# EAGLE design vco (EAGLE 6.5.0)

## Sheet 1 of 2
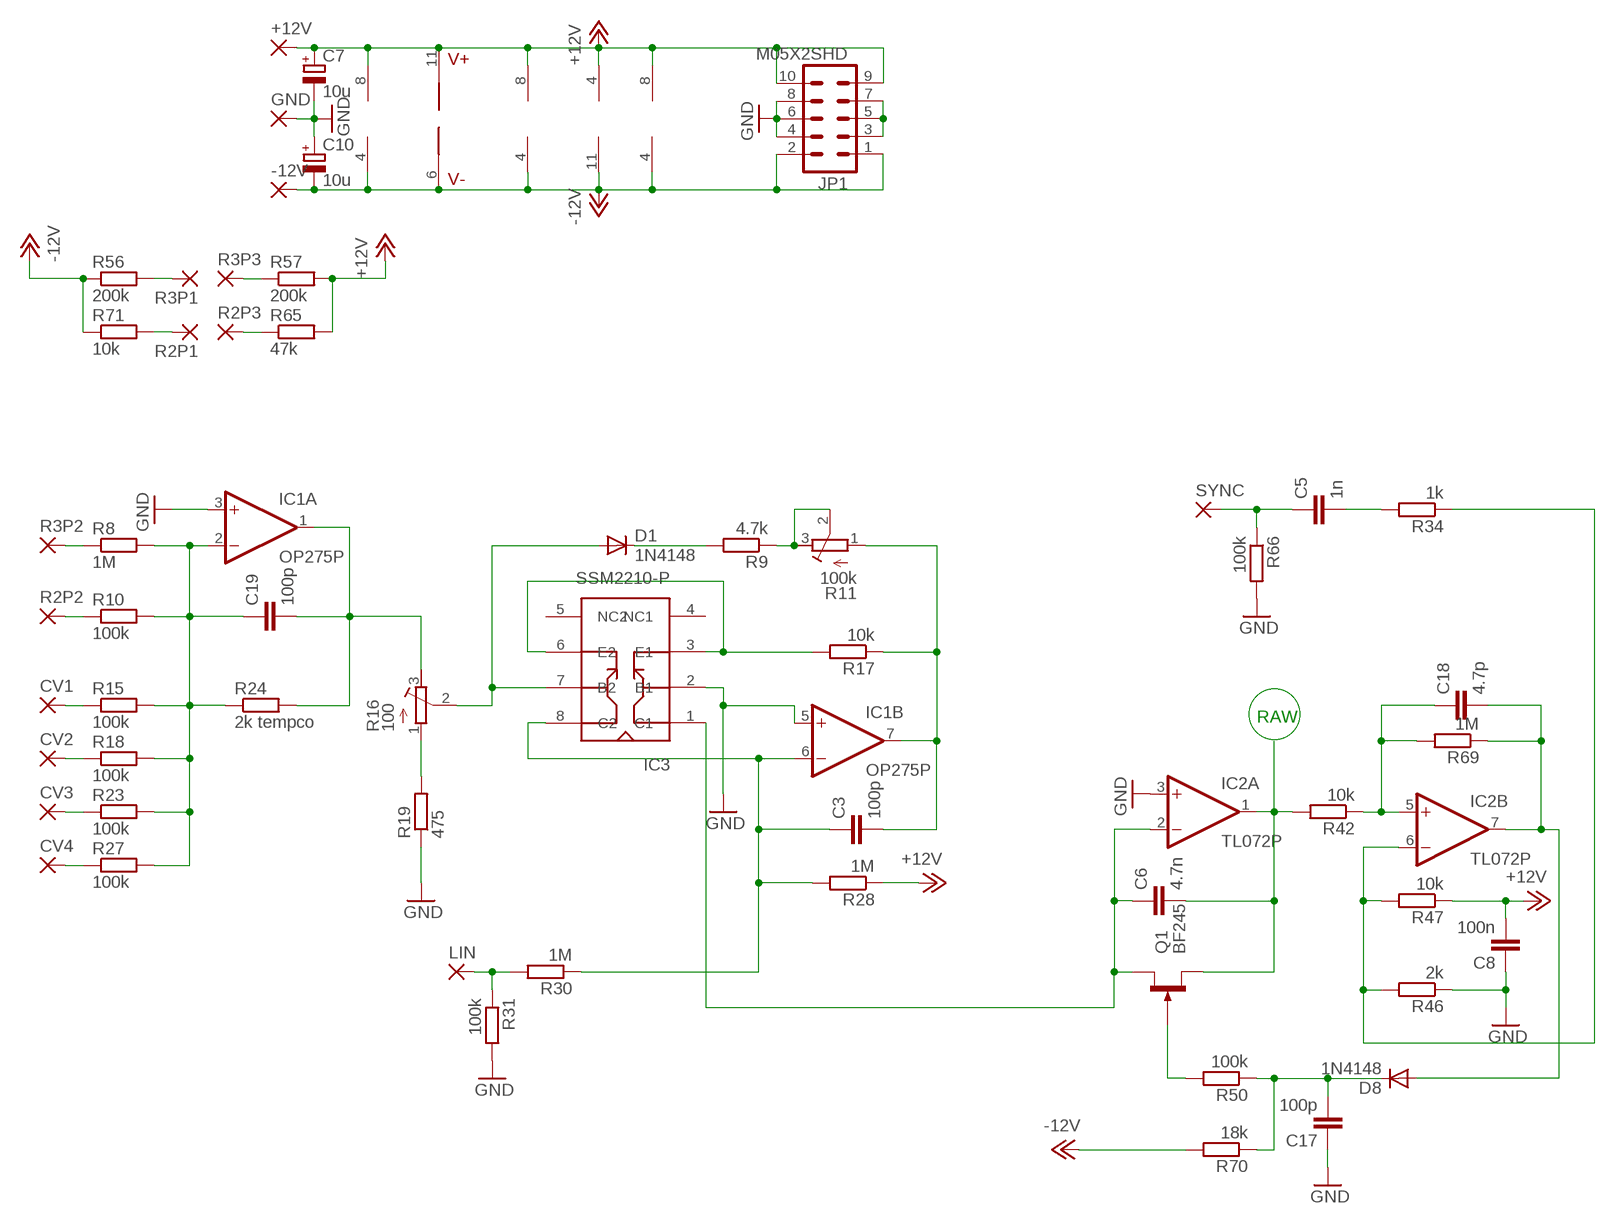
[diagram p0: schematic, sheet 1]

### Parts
+12V  2,54/1,0  [2,54/1,0]
-12V  2,54/1,0  [2,54/1,0]
C3  100p  C-EU102-043X133  [C102-043X133]
C5  1n  C-EU102-043X133  [C102-043X133]
C6  4.7n  C-EU102-043X133  [C102-043X133]
C7  10u  CPOL-EUE2.5-7  [E2,5-7]
C8  100n  C-EU102-043X133  [C102-043X133]
C10  10u  CPOL-EUE2.5-7  [E2,5-7]
C17  100p  C-EU102-043X133  [C102-043X133]
C18  4.7p  C-EU102-043X133  [C102-043X133]
C19  100p  C-EU102-043X133  [C102-043X133]
CV1  2,54/1,0  [2,54/1,0]
CV2  2,54/1,0  [2,54/1,0]
CV3  2,54/1,0  [2,54/1,0]
CV4  2,54/1,0  [2,54/1,0]
D1  1N4148  1N4148DO35-7  [DO35-7]
D8  1N4148  1N4148DO35-7  [DO35-7]
GND  2,54/1,0  [2,54/1,0]
IC1  OP275P  [DIL08]
IC2  TL072P  [DIL08]
IC3  SSM2210-P  [DIL08]
IC4  TL074P  [DIL14]
IC5  LM13700N  [DIL16]
IC6  TL072P  [DIL08]
JP1  M05X2SHD  [2X5-SHROUDED]
LIN  2,54/1,0  [2,54/1,0]
Q1  BF245  [SOT54C]
R2P1  2,54/1,0  [2,54/1,0]
R2P2  2,54/1,0  [2,54/1,0]
R2P3  2,54/1,0  [2,54/1,0]
R3P1  2,54/1,0  [2,54/1,0]
R3P2  2,54/1,0  [2,54/1,0]
R3P3  2,54/1,0  [2,54/1,0]
R8  1M  R-EU_0309/10  [0309/10]
R9  4.7k  R-EU_0309/10  [0309/10]
R10  100k  R-EU_0309/10  [0309/10]
R11  100k  R-TRIMM64W  [RTRIM64W]
R15  100k  R-EU_0309/10  [0309/10]
R16  100  R-TRIMM64W  [RTRIM64W]
R17  10k  R-EU_0309/10  [0309/10]
R18  100k  R-EU_0309/10  [0309/10]
R19  475  R-EU_0309/10  [0309/10]
R23  100k  R-EU_0309/10  [0309/10]
R24  2k tempco  R-EU_0309/12  [0309/12]
R27  100k  R-EU_0309/10  [0309/10]
R28  1M  R-EU_0309/10  [0309/10]
R30  1M  R-EU_0309/10  [0309/10]
R31  100k  R-EU_0309/10  [0309/10]
R34  1k  R-EU_0309/10  [0309/10]
R42  10k  R-EU_0309/10  [0309/10]
R46  2k  R-EU_0309/10  [0309/10]
R47  10k  R-EU_0309/10  [0309/10]
R50  100k  R-EU_0309/10  [0309/10]
R56  200k  R-EU_0309/10  [0309/10]
R57  200k  R-EU_0309/10  [0309/10]
R65  47k  R-EU_0309/10  [0309/10]
R66  100k  R-EU_0309/10  [0309/10]
R69  1M  R-EU_0309/10  [0309/10]
R70  18k  R-EU_0309/10  [0309/10]
R71  10k  R-EU_0309/10  [0309/10]
SYNC  2,54/1,0  [2,54/1,0]

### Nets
+12V: +12V.1(P) C7.+ C8.2 IC1.8(P:V+) IC2.8(P:V+) IC4.4(P:V+) IC5.11(V+) IC6.8(P:V+) JP1.9 JP1.10 R28.1 R47.1 R57.2 R65.2 ; also sheet 2
-12V: -12V.1(P) C10.- IC1.4(P:V-) IC2.4(P:V-) IC4.11(P:V-) IC5.6(V-) IC6.4(P:V-) JP1.1 JP1.2 R56.1 R70.2 R71.1 ; also sheet 2
GND: C7.- C8.1 C10.+ C17.1 GND.1(P) IC1.3(A:+IN) IC1.5(B:+IN) IC2.3(A:+IN) IC3.2(B1) JP1.4 JP1.6 JP1.8 R19.1 R31.2 R46.1 R66.2 ; also sheet 2
N$1: R3P1.1(P) R56.2
N$2: R2P1.1(P) R71.2
N$3: R2P3.1(P) R65.1
N$4: R3P3.1(P) R57.1
N$5: R3P2.1(P) R8.1
N$6: R2P2.1(P) R10.1
N$7: CV1.1(P) R15.1
N$8: CV2.1(P) R18.1
N$9: CV3.1(P) R23.1
N$10: CV4.1(P) R27.1
N$11: C19.1 IC1.2(A:-IN) R8.2 R10.2 R15.2 R18.2 R23.2 R24.1 R27.2
N$12: C19.2 IC1.1(A:OUT) R16.3(E) R24.2
N$13: Q1.G R50.2
N$14: R16.1(A) R19.2
N$15: LIN.1(P) R30.2 R31.1
N$16: C3.1 IC1.6(B:-IN) IC3.8(C2) R28.2 R30.1
N$17: C3.2 IC1.7(B:OUT) R11.1(A) R17.1
N$18: IC3.3(E1) IC3.6(E2) R17.2
N$19: C17.2 D8.C R50.1 R70.1
N$20: C6.1 IC2.2(A:-IN) IC3.1(C1) Q1.D
N$22: D1.A IC3.7(B2) R16.2(S)
N$23: D1.C R9.2
N$24: R9.1 R11.2(S) R11.3(E)
N$25: C18.1 IC2.5(B:+IN) R42.1 R69.2
N$26: C18.2 D8.A IC2.7(B:OUT) R69.1
N$27: IC2.6(B:-IN) R34.1 R46.2 R47.2
N$28: C5.2 R34.2
N$29: C5.1 R66.1 SYNC.1(P)
N$64: JP1.3 JP1.5 JP1.7
RAW: C6.2 IC2.1(A:OUT) Q1.S R42.2 ; also sheet 2
Unconnected: IC3.4(NC1) IC3.5(NC2)

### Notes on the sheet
- RAW

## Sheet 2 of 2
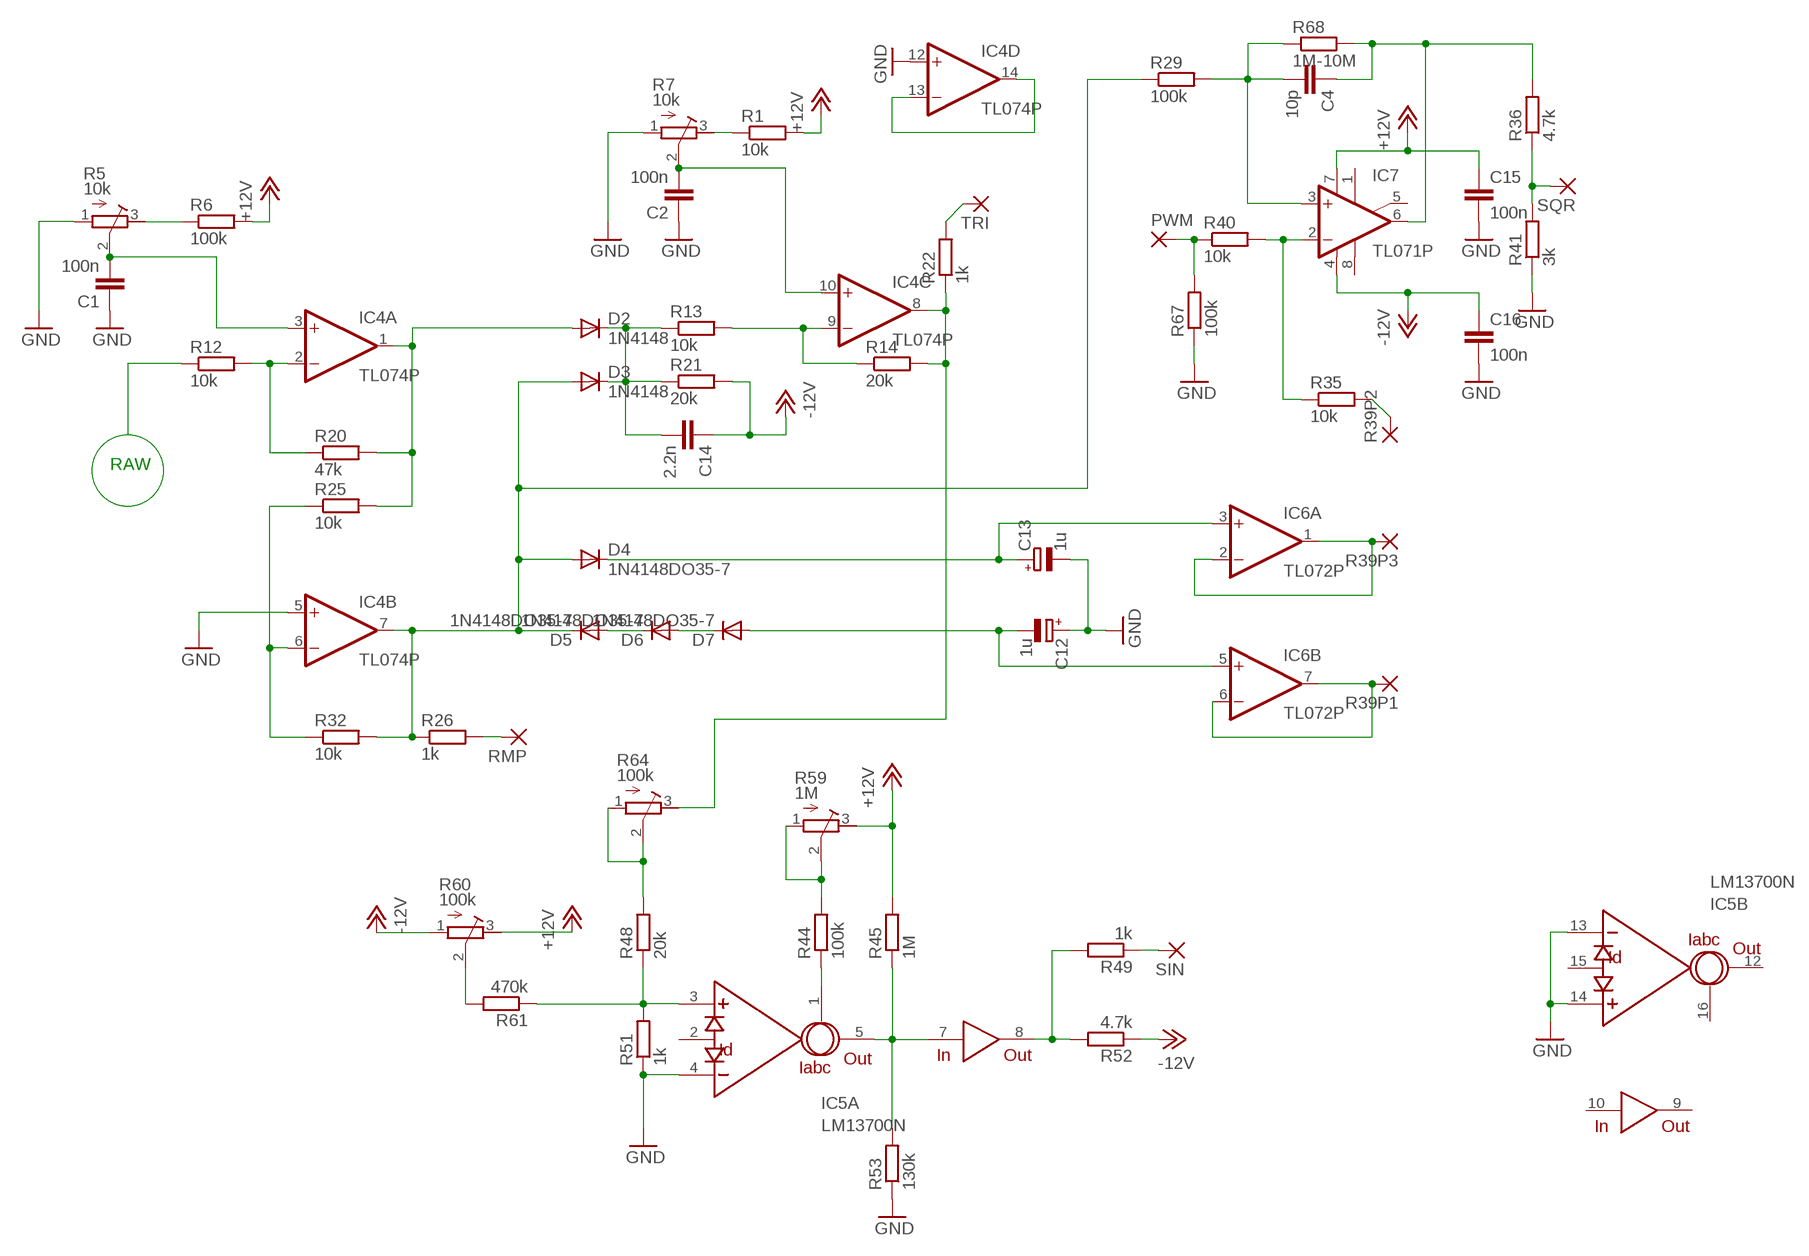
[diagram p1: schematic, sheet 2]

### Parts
C1  100n  C-EU102-043X133  [C102-043X133]
C2  100n  C-EU102-043X133  [C102-043X133]
C4  10p  C-EU102-043X133  [C102-043X133]
C12  1u  CPOL-EUE2.5-7  [E2,5-7]
C13  1u  CPOL-EUE2.5-7  [E2,5-7]
C14  2.2n  C-EU102-043X133  [C102-043X133]
C15  100n  C-EU050-035X075  [C050-035X075]
C16  100n  C-EU050-035X075  [C050-035X075]
D2  1N4148  1N4148DO35-7  [DO35-7]
D3  1N4148  1N4148DO35-7  [DO35-7]
D4  1N4148DO35-7  [DO35-7]
D5  1N4148DO35-7  [DO35-7]
D6  1N4148DO35-7  [DO35-7]
D7  1N4148DO35-7  [DO35-7]
IC7  TL071P  [DIL08]
PWM  2,54/1,0  [2,54/1,0]
R1  10k  R-EU_0309/10  [0309/10]
R5  10k  R-TRIMM64W  [RTRIM64W]
R6  100k  R-EU_0309/10  [0309/10]
R7  10k  R-TRIMM64W  [RTRIM64W]
R12  10k  R-EU_0309/10  [0309/10]
R13  10k  R-EU_0309/10  [0309/10]
R14  20k  R-EU_0309/10  [0309/10]
R20  47k  R-EU_0309/10  [0309/10]
R21  20k  R-EU_0309/10  [0309/10]
R22  1k  R-EU_0309/10  [0309/10]
R25  10k  R-EU_0309/10  [0309/10]
R26  1k  R-EU_0309/10  [0309/10]
R29  100k  R-EU_0309/10  [0309/10]
R32  10k  R-EU_0309/10  [0309/10]
R35  10k  R-EU_0309/10  [0309/10]
R36  4.7k  R-EU_0309/10  [0309/10]
R39P1  2,54/1,0  [2,54/1,0]
R39P2  2,54/1,0  [2,54/1,0]
R39P3  2,54/1,0  [2,54/1,0]
R40  10k  R-EU_0309/10  [0309/10]
R41  3k  R-EU_0309/10  [0309/10]
R44  100k  R-EU_0309/10  [0309/10]
R45  1M  R-EU_0309/10  [0309/10]
R48  20k  R-EU_0309/10  [0309/10]
R49  1k  R-EU_0309/10  [0309/10]
R51  1k  R-EU_0309/10  [0309/10]
R52  4.7k  R-EU_0309/10  [0309/10]
R53  130k  R-EU_0309/10  [0309/10]
R59  1M  R-TRIMM64W  [RTRIM64W]
R60  100k  R-TRIMM64W  [RTRIM64W]
R61  470k  R-EU_0309/10  [0309/10]
R64  100k  R-TRIMM64W  [RTRIM64W]
R67  100k  R-EU_0309/10  [0309/10]
R68  1M-10M  R-EU_0309/10  [0309/10]
RMP  2,54/1,0  [2,54/1,0]
SIN  2,54/1,0  [2,54/1,0]
SQR  2,54/1,0  [2,54/1,0]
TRI  2,54/1,0  [2,54/1,0]

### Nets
+12V: C15.1 IC7.7(V+) R1.2 R6.2 R45.2 R59.3(E) R60.3(E) ; also sheet 1
-12V: C14.1 C16.1 IC7.4(V-) R21.2 R52.1 R60.1(A) ; also sheet 1
GND: C1.1 C2.1 C12.+ C13.- C15.2 C16.2 IC4.5(B:+IN) IC4.12(D:+IN) IC5.4(A:-IN) IC5.13(B:-IN) IC5.14(B:+IN) R5.1(A) R7.1(A) R41.1 R51.1 R53.1 R67.1 ; also sheet 1
N$21: C2.2 IC4.10(C:+IN) R7.2(S)
N$30: R1.1 R7.3(E)
N$31: R26.2 RMP.1(P)
N$32: R5.3(E) R6.1
N$33: C1.2 IC4.3(A:+IN) R5.2(S)
N$34: IC4.2(A:-IN) R12.2 R20.1
N$35: D2.A IC4.1(A:OUT) R20.2 R25.2
N$36: IC4.6(B:-IN) R25.1 R32.1
N$37: IC4.13(D:-IN) IC4.14(D:OUT)
N$38: D5.A D6.C
N$39: C14.2 D2.C D3.C R13.1 R21.1
N$40: D3.A D4.A D5.C IC4.7(B:OUT) R26.1 R29.1 R32.2
N$41: IC4.9(C:-IN) R13.2 R14.1
N$42: IC4.8(C:OUT) R14.2 R22.1 R64.3(E)
N$43: R22.2 TRI.1(P)
N$44: D6.A D7.C
N$45: C13.+ D4.C IC6.3(A:+IN)
N$46: C12.- D7.A IC6.5(B:+IN)
N$47: R60.2(S) R61.2
N$48: R35.2 R39P2.1(P)
N$49: R36.1 R41.2 SQR.1(P)
N$50: IC7.2(-IN) R35.1 R40.2
N$51: PWM.1(P) R40.1 R67.2
N$52: C4.2 IC7.3(+IN) R29.2 R68.1
N$53: C4.1 IC7.6(OUT) R36.2 R68.2
N$54: IC5.3(A:+IN) R48.1 R51.2 R61.1
N$56: R48.2 R64.1(A) R64.2(S)
N$57: IC6.1(A:OUT) IC6.2(A:-IN) R39P3.1(P)
N$58: IC6.6(B:-IN) IC6.7(B:OUT) R39P1.1(P)
N$59: IC5.5(A:OUT) IC5.7(IN) R45.1 R53.2
N$60: IC5.1(A:IABC) R44.1
N$61: IC5.8(OUT) R49.2 R52.2
N$62: R44.2 R59.1(A) R59.2(S)
N$63: R49.1 SIN.1(P)
RAW: R12.1 ; also sheet 1
Unconnected: IC5.2(A:ID) IC5.9(OUT) IC5.10(IN) IC5.12(B:OUT) IC5.15(B:ID) IC5.16(B:IABC) IC7.1(ON1) IC7.5(ON2) IC7.8(OPT)

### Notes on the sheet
- RAW

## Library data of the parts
+12V -12V CV1-CV4 GND LIN PWM R2P1-R2P3 R3P1-R3P3 R39P1-R39P3 RMP SIN SQR SYNC TRI = wirepad:2,54/1,0: THROUGH-HOLE PAD
C1-C6 C8 C14-C19 = rcl:C-EU: CAPACITOR, European symbol
C7 C10 C12 C13 = rcl:CPOL-EU: POLARIZED CAPACITOR, European symbol
D1-D8 = diode:1N4148: DIODE
IC1 = linear:OP275: Dual Very Low Noise Precision Operational Amplifier Source: http://www.analog.com/static/imported-files/data_sheets/OP270.pdf
IC2 IC6 = linear:TL072: OP AMP
IC3 = cavalier:SSM2210
IC4 = linear:TL074: OP AMP
IC5 = synthdiy:LM13700: National Dual OTA with buffers.
IC7 = linear:TL071: OP AMP
JP1 = SparkFun:M05X2: Header 5x2 Standard 10-pin dual row 0.1" header. Commonly used with AVR-ISP. Use with Spark Fun Electronics SKU: PRT-00778
Q1 = transistor-small-signal:BF245: N-CHANNEL FET http://www.onsemi.com/pub/Collateral/BF245A-D.PDF
R1 R6 R8-R10 R12-R15 R17-R32 R34-R36 R40-R42 R44-R53 R56 R57 R61 R65-R71 = rcl:R-EU_: RESISTOR, European symbol
R5 R7 R11 R16 R59 R60 R64 = rcl:R-TRIMM: Trimm resistor

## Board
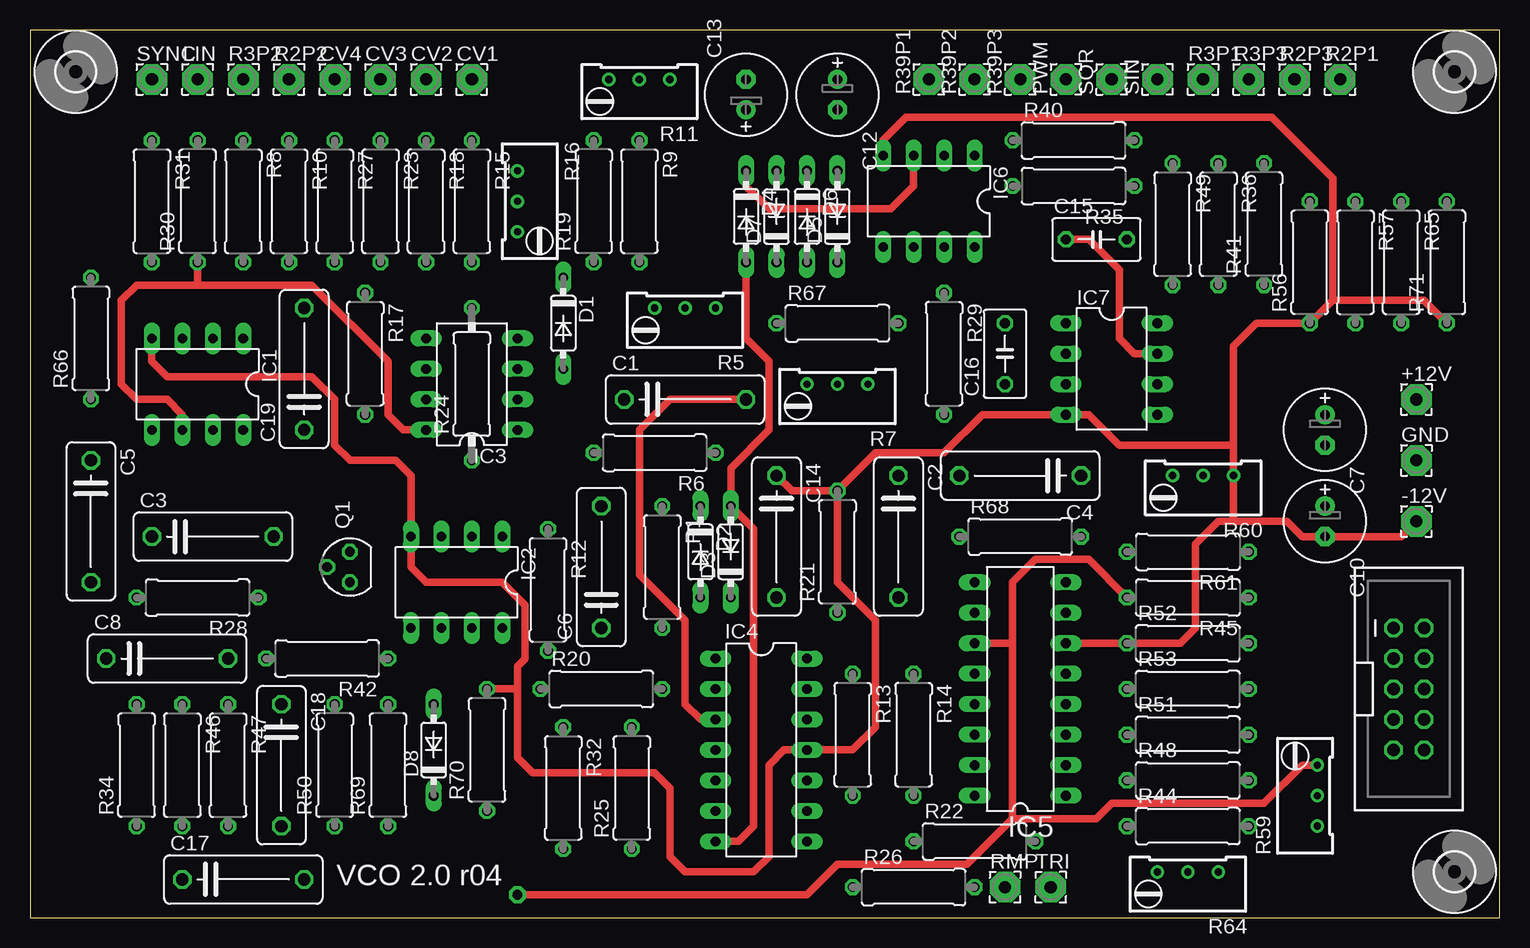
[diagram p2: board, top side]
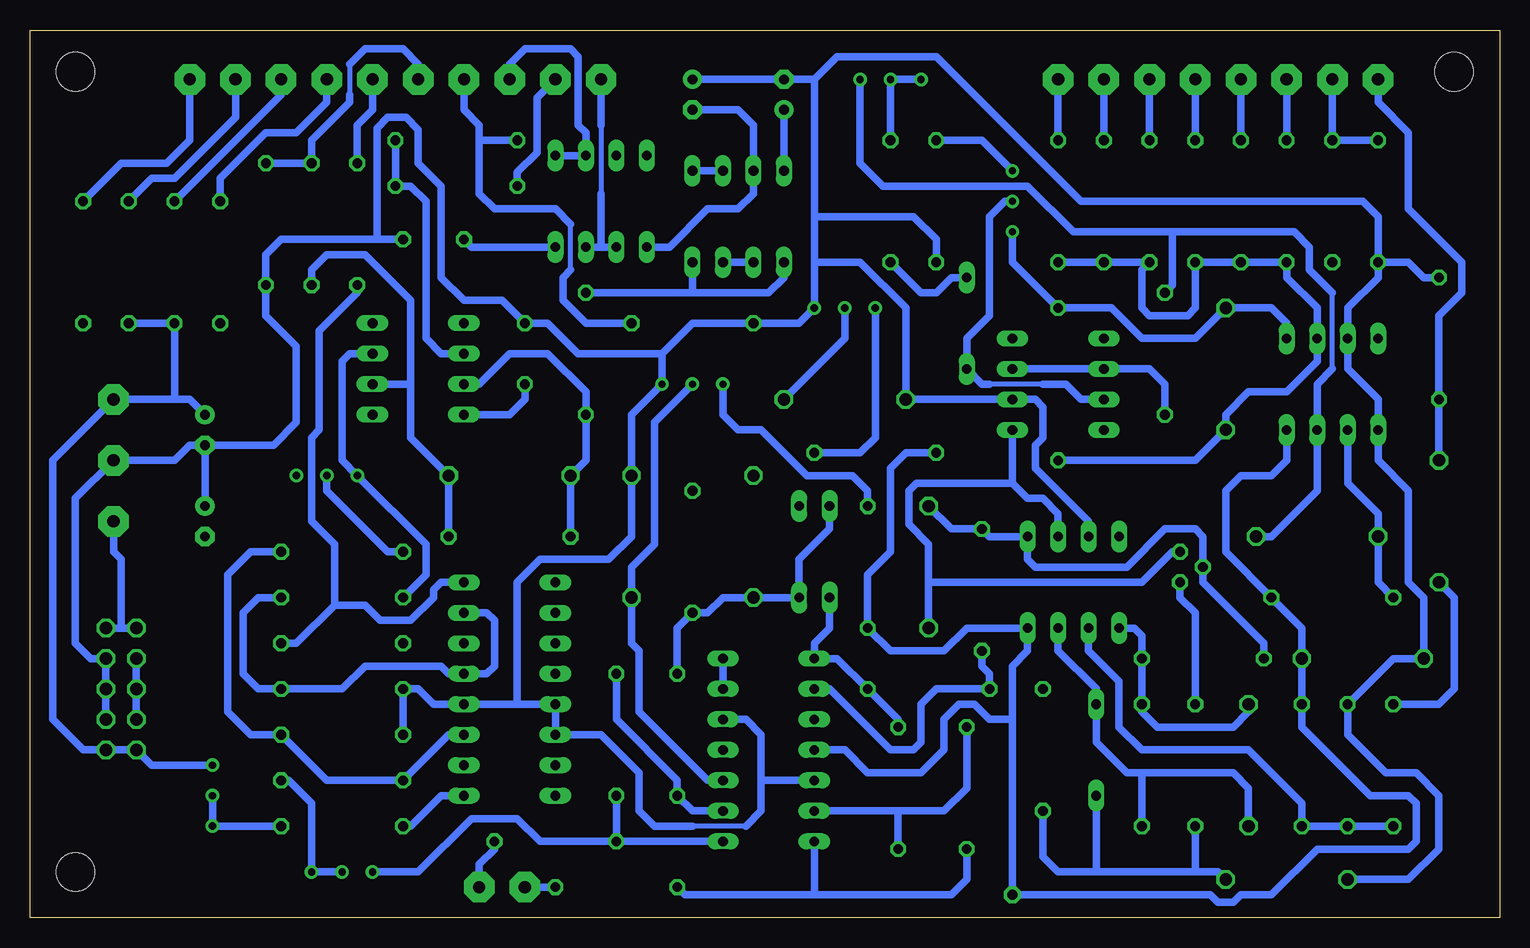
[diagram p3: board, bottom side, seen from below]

Size 122.53 x 73.97 mm. Coordinates in mm from the lower left corner, seen from the top.
Outline: 0,0 122.53,0 122.53,73.97 0,73.97 0,0
Copper layers (1*16): Top 0.035mm / dielectric 1.5mm / Bottom 0.035mm
Design rules "default": minimum track width 10mil, minimum drill 24mil, track to track 8mil, track to pad 8mil, pad to pad 8mil, via to via 8mil, smd to smd 8mil, copper to edge 40mil, drill to drill 8mil, minimum pad ring 10mil, minimum via ring 8mil, stop-mask expansion 4mil, vias tented up to drill 0mil, thermal gap 10mil

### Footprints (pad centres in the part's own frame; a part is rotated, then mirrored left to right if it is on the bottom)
2,54/1,0 = drill 1.016 pad 2.54 octagon: 1 0,0
C102-043X133 = drill 1.016 octagon: 1 -5.08,0; 2 5.08,0
E2,5-7 = drill 0.813 pad 1.6: + -1.27,0 | drill 0.813 pad 1.6 octagon: - 1.27,0
C050-035X075 = drill 0.813 octagon: 1 -2.54,0; 2 2.54,0
DO35-7 = drill 0.813 long: A 3.81,0; C -3.81,0
DIL08 = drill 0.813 pad 1.27 long: 1 -3.81,-3.81; 2 -1.27,-3.81; 3 1.27,-3.81; 4 3.81,-3.81; 5 3.81,3.81; 6 1.27,3.81; 7 -1.27,3.81; 8 -3.81,3.81
DIL14 = drill 0.813 long: 1 -7.62,-3.81; 2 -5.08,-3.81; 3 -2.54,-3.81; 4 0,-3.81; 5 2.54,-3.81; 6 5.08,-3.81; 7 7.62,-3.81; 8 7.62,3.81; 9 5.08,3.81; 10 2.54,3.81; 11 0,3.81; 12 -2.54,3.81; 13 -5.08,3.81; 14 -7.62,3.81
DIL16 = drill 0.813 long: 1 -8.89,-3.81; 2 -6.35,-3.81; 3 -3.81,-3.81; 4 -1.27,-3.81; 5 1.27,-3.81; 6 3.81,-3.81; 7 6.35,-3.81; 8 8.89,-3.81; 9 8.89,3.81; 10 6.35,3.81; 11 3.81,3.81; 12 1.27,3.81; 13 -1.27,3.81; 14 -3.81,3.81; 15 -6.35,3.81; 16 -8.89,3.81
2X5-SHROUDED = drill 1.016 octagon: 1 -1.27,5.08; 2 1.27,5.08; 3 -1.27,2.54; 4 1.27,2.54; 5 -1.27,0; 6 1.27,0; 7 -1.27,-2.54; 8 1.27,-2.54; 9 -1.27,-5.08; 10 1.27,-5.08
SOT54C = drill 0.813 octagon: D 1.27,0; G -1.27,0; S 0,1.905
0309/10 = drill 0.813 octagon: 1 -5.08,0; 2 5.08,0
RTRIM64W = drill 0.61: 1 1.27,-2.54; 2 1.27,0; 3 1.27,2.54
0309/12 = drill 0.813 octagon: 1 -6.35,0; 2 6.35,0
3,2 = hole 3.2: 0,0

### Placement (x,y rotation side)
+12V  115.57,43.18 0 top
-12V  115.57,33.02 0 top
C1  54.61,43.18 0 top
C2  72.39,31.75 270 top
C3  15.24,31.75 0 top
C4  82.55,36.83 180 top
C5  5.08,33.02 270 top
C6  47.62,29.21 90 top
C7  107.95,40.64 270 top
C8  11.43,21.59 0 top
C10  107.95,33.02 270 top
C12  67.31,68.58 270 top
C13  59.69,68.58 90 top
C14  62.23,31.75 270 top
C15  88.9,56.52 0 top
C16  81.28,46.99 90 top
C17  17.78,3.17 0 top
C18  20.95,12.7 270 top
C19  22.86,45.72 90 top
CV1  36.83,69.85 0 top
CV2  33.02,69.85 0 top
CV3  29.21,69.85 0 top
CV4  25.4,69.85 0 top
D1  44.45,49.53 270 top
D2  55.88,30.48 270 top
D3  58.42,30.48 90 top
D4  59.69,58.42 270 top
D5  67.31,58.42 90 top
D6  64.77,58.42 270 top
D7  62.23,58.42 90 top
D8  33.66,13.97 90 top
GND  115.57,38.1 0 top
IC1  13.97,44.45 180 top
IC2  35.56,27.94 180 top
IC3  36.83,44.45 90 top
IC4  60.96,13.97 270 top
IC5  82.55,19.05 90 top
IC6  74.93,59.69 180 top
IC7  90.17,45.72 270 top
JP1  114.94,19.05 0 top
LIN  13.97,69.85 0 top
PWM  86.36,69.85 90 top
Q1  26.67,29.21 90 top
R1  52.7,29.21 270 top
R2P1  109.22,69.85 0 top
R2P2  21.59,69.85 0 top
R2P3  105.41,69.85 0 top
R3P1  97.79,69.85 0 top
R3P2  17.78,69.85 0 top
R3P3  101.6,69.85 0 top
R5  54.61,49.53 90 top
R6  52.07,38.73 180 top
R7  67.31,43.18 90 top
R8  17.78,59.69 270 top
R9  50.8,59.69 270 top
R10  21.59,59.69 270 top
R11  50.8,68.58 90 top
R12  43.18,27.3 270 top
R13  68.58,15.24 270 top
R14  73.66,15.24 270 top
R15  36.83,59.69 270 top
R16  41.91,59.69 180 top
R17  27.94,46.99 270 top
R18  33.02,59.69 270 top
R19  46.99,59.69 90 top
R20  47.62,19.05 0 top
R21  67.31,30.48 90 top
R22  78.74,6.35 0 top
R23  29.21,59.69 270 top
R24  36.83,44.45 90 top
R25  50.16,10.79 90 top
R26  73.66,2.54 0 top
R27  25.4,59.69 270 top
R28  13.97,26.67 180 top
R29  76.2,46.99 270 top
R30  13.97,59.69 90 top
R31  10.16,59.69 270 top
R32  44.45,10.79 270 top
R34  8.89,12.7 90 top
R35  87,60.96 180 top
R36  99.06,57.78 270 top
R39P1  74.93,69.85 90 top
R39P2  78.74,69.85 90 top
R39P3  82.55,69.85 90 top
R40  87,64.77 0 top
R41  102.87,57.78 90 top
R42  24.77,21.59 180 top
R44  96.52,7.62 0 top
R45  96.52,26.67 180 top
R46  12.7,12.7 270 top
R47  16.51,12.7 270 top
R48  96.52,11.43 0 top
R49  95.25,57.78 270 top
R50  25.4,12.7 90 top
R51  96.52,15.24 0 top
R52  96.52,22.86 0 top
R53  96.52,19.05 0 top
R56  106.68,54.61 90 top
R57  110.49,54.61 270 top
R59  106.05,10.16 0 top
R60  97.79,35.56 90 top
R61  96.52,30.48 180 top
R64  96.52,2.54 90 top
R65  114.3,54.61 270 top
R66  5.08,48.26 90 top
R67  67.31,49.53 0 top
R68  82.55,31.75 0 top
R69  29.84,12.7 90 top
R70  38.1,13.97 90 top
R71  118.11,54.61 90 top
RMP  81.28,2.54 0 top
SIN  93.98,69.85 90 top
SQR  90.17,69.85 90 top
SYNC  10.16,69.85 0 top
TRI  85.09,2.54 0 top
U$1  [3,2]  3.81,70.48 0 top
U$2  [3,2]  118.75,70.48 0 top
U$3  [3,2]  118.75,3.81 0 top

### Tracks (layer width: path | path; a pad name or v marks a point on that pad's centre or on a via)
+12V  (via drill 0.8 pad 1.42)
  Top 0.61: 81.92,8.26 78.11,4.45 67.31,4.45 64.77,1.91 v40.64,1.91 | 81.92,22.86 81.92,8.26 | 81.92,8.26 88.9,8.26 90.17,9.53 102.87,9.53 106.05,12.7 R59.3 | IC5.11 81.92,22.86 | 81.92,22.86 81.92,27.94 83.82,29.84 88.27,29.84 R45.2 | C15.1 88.27,56.52 90.81,53.98 90.81,48.26 92.08,46.99 IC7.7
  Bottom 0.61: 110.49,43.18 +12V.1 120.65,38.1 120.65,16.51 118.11,13.97 JP1.10 JP1.9 112.39,12.7 R59.3 | 110.49,43.18 109.22,43.18 C7.+ | IC1.8 17.78,38.1 19.05,36.83 21.59,36.83 22.86,35.56 22.86,30.48 R28.1 16.51,24.13 C8.2 R47.1 16.51,15.88 10.79,10.16 7.62,10.16 6.99,9.53 6.99,6.35 7.62,5.71 15.24,5.71 19.05,1.91 21.59,1.91 22.23,1.27 23.5,1.27 24.13,1.91 v40.64,1.91 40.64,16.51 | R45.2 89.53,28.57 89.53,31.11 R60.3 96.52,38.1 96.52,46.35 95.89,46.99 IC7.7 | IC6.8 85.72,55.88 C15.1 | 40.64,16.51 40.64,20.95 39.37,22.23 IC2.8 44.45,24.13 46.35,22.23 50.8,22.23 R1.2 52.7,28.57 50.8,30.48 50.8,37.47 49.53,38.73 R6.2 | R65.2 R57.2 110.49,43.18 | IC4.4 54.61,13.97 52.7,12.06 48.26,12.06 46.35,13.97 46.35,16.51 45.09,17.78 43.81,17.78 42.55,16.51 40.64,16.51
-12V
  Top 0.61: 100.33,39.37 R60.1 100.33,33.02 | 100.33,39.37 90.81,39.37 88.27,41.91 IC7.4 79.38,41.91 76.2,38.73 70.48,38.73 R21.2 | IC1.4 10.16,46.35 11.43,45.09 23.5,45.09 25.4,43.18 25.4,39.37 26.67,38.1 30.48,38.1 31.75,36.83 IC2.4 31.75,29.21 33.02,27.94 39.37,27.94 41.27,26.04 41.27,21.59 40.64,20.95 40.64,19.05 | C14.1 63.5,35.56 R21.2 | R21.2 67.31,27.94 70.48,24.77 70.48,15.88 68.58,13.97 IC4.11 62.87,13.97 61.59,12.7 61.59,5.08 60.33,3.81 54.61,3.81 53.34,5.08 53.34,10.79 52.07,12.06 41.91,12.06 40.64,13.34 40.64,19.05 | 100.33,33.02 99.06,33.02 97.16,31.11 97.16,24.13 95.89,22.86 R52.1 IC5.6 | 100.33,33.02 104.78,33.02 106.05,31.75 C10.- 114.3,31.75 -12V.1 | 100.33,39.37 100.33,47.62 102.23,49.53 R56.1 108.58,51.44 | 108.58,51.44 108.58,61.59 103.5,66.67 73.03,66.67 71.12,64.77 IC6.4 | 108.58,51.44 116.2,51.44 R71.1 | R70.2 40.64,19.05
  Bottom 0.61: IC7.4 82.55,41.91 81.28,43.18 C16.1 | JP1.2 114.94,24.13 | JP1.1 114.94,24.13 | 114.94,24.13 114.94,29.84 115.57,30.48 -12V.1
GND
  Bottom 0.406: 62.87,7.62 67.31,7.62
  Bottom 0.61: C7.- 109.22,39.37 110.49,38.1 GND.1 118.75,34.92 118.75,22.86 117.47,21.59 JP1.4 JP1.6 JP1.8 | 69.85,46.99 R7.1 72.39,41.91 C2.1 72.39,31.75 74.3,29.84 80.01,29.84 81.92,27.94 81.92,17.78 | 69.85,46.99 67.31,49.53 R67.1 58.42,49.53 R5.1 57.15,54.61 | 57.15,54.61 57.15,58.42 | 57.15,58.42 57.15,69.85 | 58.42,69.85 C13.- | C13.- C12.+ | R19.1 46.99,56.52 48.9,58.42 57.15,58.42 | 57.15,54.61 53.34,54.61 49.53,50.8 C1.1 IC3.2 38.73,43.18 38.1,42.55 38.1,40.01 38.73,39.37 38.73,37.47 34.29,33.02 IC2.3 | R66.2 6.35,53.34 7.62,54.61 R31.2 | R31.2 10.16,58.42 11.43,59.69 34.92,59.69 46.99,71.75 55.24,71.75 57.15,69.85 | R31.2 10.16,53.34 12.7,50.8 IC1.3 12.7,45.72 10.16,43.18 IC1.5 10.16,38.1 7.62,35.56 7.62,27.94 6.35,26.67 C8.1 8.89,21.59 R46.1 12.7,15.24 9.53,12.06 6.99,12.06 5.08,10.16 5.08,5.71 7.62,3.17 C17.1 | IC4.5 61.59,11.43 | 61.59,11.43 61.59,15.24 62.87,16.51 IC4.12 | 81.92,17.78 IC5.13 IC5.14 74.93,15.24 71.75,12.06 71.75,8.89 70.48,7.62 67.31,7.62 | 81.92,17.78 IC5.4 88.9,17.78 90.17,19.05 R53.1 R51.1 | 61.59,11.43 61.59,8.89 62.87,7.62 | 57.15,69.85 C13.- | 93.6,56.52 101.6,56.52 102.87,55.24 R41.1 102.87,50.16 100.33,47.62 100.33,41.27 102.23,39.37 C7.- | C10.+ C7.- | 69.85,46.99 76.83,46.99 79.38,49.53 C16.2 83.19,51.44 86.36,51.44 88.27,53.34 88.27,60.96 90.17,62.87 90.17,65.66 91.19,66.67 92.71,66.67 93.6,65.79 93.6,56.52 | C15.2 93.6,56.52
N$1
  Bottom 0.61: R3P1.1 97.79,67.94 100.33,65.41 102.87,65.41 106.68,61.59 R56.2
N$2
  Bottom 0.61: R2P1.1 109.22,64.77 111.12,62.87 114.94,62.87 R71.2
N$3
  Bottom 0.61: R2P3.1 105.41,66.67 110.49,61.59 112.39,61.59 R65.1
N$4
  Bottom 0.61: R3P3.1 101.6,68.58 R57.1
N$5
  Bottom 0.61: R8.1 R3P2.1
N$6
  Bottom 0.61: R10.1 R2P2.1
N$7
  Bottom 0.61: R15.1 CV1.1
N$8
  Bottom 0.61: R18.1 CV2.1
N$9
  Bottom 0.61: R23.1 CV3.1
N$10
  Bottom 0.61: R27.1 CV4.1
N$11
  Bottom 0.61: R15.2 R18.2 R23.2 29.84,53.98 29.84,50.8 29.21,50.16 26.04,50.16 25.4,50.8 R27.2 R10.2 R8.2 17.78,53.34 15.24,50.8 IC1.2 15.24,46.35 17.78,43.81 20.95,43.81 22.86,41.91 C19.1 25.4,38.1 R24.1
N$12
  Bottom 0.61: IC1.1 17.78,49.53 19.05,50.8 C19.2 25.4,48.26 29.84,48.26 32.38,50.8 R24.2 40.64,54.61 R16.3
N$13
  Bottom 0.61: R50.2 25.4,25.4 26.67,26.67 Q1.G
N$14
  Bottom 0.61: R16.1 43.18,64.77 R19.2
N$15
  Bottom 0.61: R31.1 R30.2 LIN.1
N$16
  Top 0.61: R30.1 13.97,52.7 | 13.97,52.7 8.89,52.7 7.62,51.44 7.62,44.45 8.89,43.18 11.43,43.18 12.7,41.91 IC1.6 | IC3.8 31.11,40.64 29.84,41.91 29.84,46.35 23.5,52.7 13.97,52.7
  Bottom 0.61: R28.2 10.16,27.94 C3.1 10.16,33.66 12.7,36.2 IC1.6
N$17
  Bottom 0.406: 13.97,45.72 13.97,52.07
  Bottom 0.61: C3.2 19.05,31.75 15.24,35.56 IC1.7 15.24,44.45 13.97,45.72 | 13.97,52.07 15.88,53.98 15.88,55.88 17.14,57.15 27.3,57.15 | R17.1 27.3,52.7 27.3,57.15 | 27.3,57.15 35.56,57.15 39.37,60.96 51.44,60.96 53.34,62.87 R11.1
N$18
  Bottom 0.61: IC3.3 IC3.6 29.21,45.72 27.94,44.45 R17.2
N$19
  Bottom 0.61: C17.2 23.5,3.81 25.4,3.81 | 25.4,3.81 33.66,3.81 | 33.66,3.81 36.83,3.81 38.1,5.08 R70.1 | D8.C 33.66,3.81 | R50.1 25.4,3.81
N$20
  Bottom 0.61: 47.62,27.94 47.62,31.11 49.28,32.77 49.28,35.56 48.64,36.2 40.64,36.2 | 47.62,27.94 C6.1 | IC3.1 40.64,36.2 | 47.62,27.94 29.84,27.94 27.3,30.48 Q1.D | IC2.2 36.83,33.66 38.1,34.92 39.37,34.92 40.64,36.2
N$21
  Bottom 0.61: IC4.10 66.04,11.43 71.75,17.14 71.75,22.23 72.39,22.86 C2.2 72.39,29.21 70.48,31.11 70.48,41.27 R7.2
N$22
  Bottom 0.406: 38.1,44.45 42.55,44.45
  Bottom 0.61: IC3.7 34.92,43.18 36.2,44.45 38.1,44.45 | 42.55,44.45 43.18,44.45 D1.A 44.45,48.26 42.55,50.16 42.55,58.42 41.27,59.69 R16.2
N$23
  Bottom 0.61: R9.2 48.26,52.07 46.99,52.07 45.72,53.34 D1.C
N$24
  Bottom 0.61: R9.1 R11.2 R11.3
N$25
  Bottom 0.61: C18.1 20.95,17.14 22.23,15.88 28.57,15.88 29.84,17.14 R69.2 R42.1 29.84,23.5 30.48,24.13 IC2.5
N$26
  Bottom 0.61: C18.2 20.95,10.79 22.23,12.06 29.84,12.06 | 29.84,12.06 31.11,12.06 33.66,14.61 D8.A 33.66,19.05 36.83,22.23 IC2.7 | R69.1 29.84,12.06
N$27
  Bottom 0.61: R34.1 R46.2 R47.2 16.51,9.53 20.95,13.97 29.84,13.97 31.75,15.88 31.75,19.68 34.29,22.23 IC2.6
N$28
  Bottom 0.61: C5.2 3.81,26.67 3.81,19.05 5.08,17.78 R34.2
N$29
  Bottom 0.61: C5.1 R66.1 5.08,50.16 3.17,52.07 3.17,54.61 7.62,59.05 7.62,65.41 10.16,67.94 SYNC.1
N$30
  Bottom 0.61: R1.1 52.7,35.56 53.98,36.83 57.78,36.83 61.59,40.64 63.5,40.64 64.77,41.91 R7.3
N$31
  Bottom 0.61: RMP.1 R26.2
N$32
  Bottom 0.61: R5.3 52.07,40.01 53.34,38.73 R6.1
N$33
  Top 0.61: IC4.3 55.88,16.51 54.61,17.78 54.61,24.77 50.8,28.57 50.8,40.64 53.34,43.18 C1.2
  Bottom 0.61: R5.2 54.61,48.26 C1.2
N$34
  Bottom 0.61: R12.2 43.18,20.95 42.55,20.32 R20.1 46.99,19.05 48.26,17.78 48.26,14.61 48.9,13.97 50.8,13.97 55.88,19.05 IC4.2
N$35
  Bottom 0.61: D2.A 55.88,24.13 57.15,22.86 IC4.1 55.24,21.59 R20.2 50.16,16.51 R25.2
N$36
  Bottom 0.61: IC4.6 50.16,8.89 | 50.16,8.89 46.35,8.89 44.45,10.79 R32.1 | R25.1 50.16,8.89
N$37
  Bottom 0.61: IC4.13 IC4.14
N$38
  Bottom 0.61: D5.A D6.C
N$39
  Bottom 0.61: R13.1 68.58,24.13 R21.1 66.04,25.4 64.77,26.67 C14.2 D3.C 58.42,29.84 55.88,32.38 D2.C
N$40
  Top 0.61: IC4.7 59.05,6.35 60.33,7.62 60.33,32.38 D3.A 58.42,37.47 61.59,40.64 61.59,46.35 59.69,48.26 D4.A
  Bottom 0.61: 57.15,1.91 45.72,1.91 44.45,3.17 R32.2 | 57.15,1.91 67.94,1.91 R26.1 | IC4.7 57.15,1.91 | R29.1 67.31,52.07 | 67.31,52.07 60.96,52.07 59.69,53.34 D4.A | D5.C 67.31,52.07
N$41
  Bottom 0.61: IC4.9 67.31,8.89 R13.2 68.58,11.43 73.66,16.51 R14.1
N$42
  Bottom 0.61: R64.3 90.17,3.81 85.72,8.26 81.92,8.26 80.01,6.35 R22.1 | R22.1 R14.2 | IC4.8 R22.1
N$43
  Bottom 0.61: R22.2 83.82,5.71 85.09,4.45 TRI.1
N$44
  Bottom 0.61: D6.A D7.C
N$45
  Top 0.61: IC6.3 73.66,60.96 71.75,59.05 61.59,59.05 59.69,60.96 D4.C
  Bottom 0.61: C13.+ D4.C
N$46
  Bottom 0.61: IC6.5 69.22,55.88 66.04,59.05 63.5,59.05 62.23,60.33 D7.A 62.23,66.04 63.5,67.31 C12.-
N$47
  Bottom 0.61: R60.2 97.79,35.56 92.71,30.48 R61.2
N$48
  Bottom 0.61: R35.2 81.92,62.1 80.26,63.75 80.26,68.33 R39P2.1
N$49
  Bottom 0.406: 95.89,71.12 95.89,68.58
  Bottom 0.61: R41.2 R36.1 99.06,64.77 95.89,67.94 95.89,68.58 | SQR.1 90.17,71.12 91.44,72.39 94.61,72.39 95.89,71.12
N$50
  Bottom 0.61: R40.2 R35.1 90.81,60.96 89.53,59.69 89.53,48.26 88.27,46.99 IC7.2
N$51
  Bottom 0.406: 77.47,53.98 77.47,57.78
  Bottom 0.61: R67.2 76.2,49.53 78.11,51.44 78.11,53.34 77.47,53.98 | 77.47,57.78 78.74,59.05 83.82,59.05 85.09,60.33 85.09,64.77 | 85.09,64.77 85.09,66.04 86.36,67.31 PWM.1 | R40.1 85.09,64.77
N$52
  Bottom 0.61: IC7.3 85.09,44.45 82.55,46.99 79.38,46.99 76.2,43.81 R29.2 76.2,38.1 C4.2 R68.1
N$53
  Bottom 0.61: R68.2 C4.1 90.81,40.01 90.81,44.45 | R36.2 99.06,53.98 97.79,55.24 94.61,55.24 90.81,51.44 90.81,44.45 | IC7.6 90.81,44.45
N$54
  Bottom 0.61: IC5.3 87.63,15.24 R48.1 97.79,11.43 R51.2 104.14,15.24 106.05,17.14 106.05,28.57 104.14,30.48 R61.1
N$56
  Bottom 0.61: R64.2 R64.1 99.06,9.53 100.97,11.43 R48.2
N$57
  Bottom 0.61: R39P3.1 82.55,71.12 81.28,72.39 77.47,72.39 76.83,71.75 76.83,66.04 76.2,65.41 IC6.2 IC6.1
N$58
  Bottom 0.406: 74.93,66.04 74.93,60.33
  Bottom 0.61: IC6.7 74.93,55.88 | 74.93,55.88 IC6.6 | R39P1.1 74.93,66.04 | 74.93,60.33 74.93,55.88
N$59
  Bottom 0.61: R45.1 103.5,26.67 104.78,25.4 104.78,20.32 103.5,19.05 R53.2 96.52,19.05 94.61,20.95 88.27,20.95 87.63,20.32 IC5.5 84.45,20.32 83.82,20.95 83.82,24.77 84.45,25.4 IC5.7
N$60
  Bottom 0.61: R44.1 90.81,7.62 88.27,10.16 IC5.1
N$61
  Bottom 0.61: R52.2 100.33,22.86 97.16,26.04 | IC5.8 88.27,27.94 88.9,27.3 88.9,26.67 90.81,24.77 93.34,24.77 94.61,26.04 97.16,26.04 | 97.16,26.04 97.16,31.11 99.06,33.02 99.06,40.01 98.42,40.64 98.42,48.9 95.25,52.07 R49.2
N$62
  Bottom 0.61: R59.2 R59.1 R44.2
N$63
  Bottom 0.61: SIN.1 93.98,67.31 95.25,66.04 R49.1
N$64
  Bottom 0.61: JP1.7 JP1.5 JP1.3
RAW
  Bottom 0.61: R42.2 19.68,22.86 24.77,27.94 Q1.S 24.77,31.75 25.4,32.38 27.94,32.38 31.11,29.21 38.73,29.21 39.37,29.84 IC2.1 42.55,31.75 R12.1 45.72,32.38 C6.2

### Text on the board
tNames: VCO 2.0 r04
